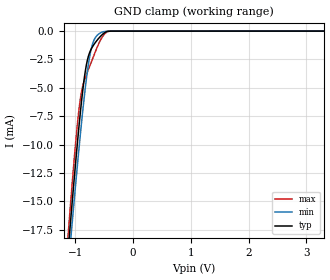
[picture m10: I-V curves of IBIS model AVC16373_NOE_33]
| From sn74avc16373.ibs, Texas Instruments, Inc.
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[Model]   AVC16373_NOE_33
Model_type  Input
Vinl=0.8
Vinh=2
| variable   typ   min   max
C_comp   1.84pF   1.29pF   2.54pF
[Temperature Range]   40   100   -40
| Ambient temperature   25   85   -40
[Voltage range]   3.3   3   3.6
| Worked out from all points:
|   GND clamp passes 1 mA (typ) near -0.65 V on its own axis
[GND Clamp]
| AVC16373_NOE_33
|   Voltage   I(typ)   I(min)   I(max)
-3.3V     -168.4mA   -162.8mA   -178.2mA
-1.12V    -19.01mA   -20.68mA   -17.58mA
-1.1V     -17.78mA   -19.5mA    -16.27mA
-1.065V   -15.65mA   -17.45mA   -14.03mA
-985mV    -10.97mA   -12.91mA   -9.257mA
-930mV    -7.991mA   -9.944mA   -6.576mA
-885mV    -5.791mA   -7.647mA   -5.114mA
-825mV    -3.443mA   -4.871mA   -4.055mA
-715mV    -1.48mA    -1.36mA    -2.619mA
-570mV    -489.8uA   -169.9uA   -837.3uA
-370mV    -4.236uA   -3.71uA    -3.93uA
3.3V      214.2pA    699.5pA    13.28pA
